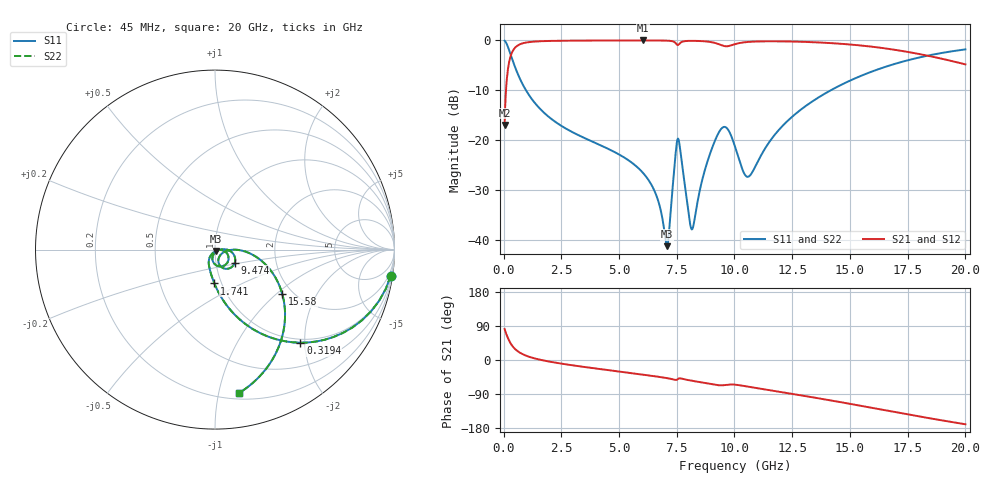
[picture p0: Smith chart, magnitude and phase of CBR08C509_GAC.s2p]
! S-parameter model data by Modelithics Inc.  support@modelithics.com 813-866-6335  Tampa FL USA
! S-Parameter data specifications:
! Substrate: 20-mil Rogers 4350B, substrate thickness, H=0.508mm, Dielectric constant, Er=3.75
! PCB Mounting Pad Footprint: Pad width, PadW=1.45mm , Pad length, PadL=1mm , Pad gap, PadG (edge-to-edge)=0.6mm , Reference planes=2.6mm apart
#  GHz  S  MA  R 50
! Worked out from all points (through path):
!   801 points, 45 MHz to 20 GHz, reference 50 ohm
!   highest |S21| = -0.04 dB at 6.032 GHz (marker M1); lowest = -17.0 dB at 45 MHz (marker M2)
!   group delay of S21, straight-line fit = 25.7 ps
!   lowest |S11| = -41.3 dB at 7.079 GHz (marker M3), VSWR 1.02, Z = 50.4 - j0.777 ohm
!   |S11| at or under -10 dB: 965.8 MHz to 14.18 GHz (13.22 GHz wide, 175 % of centre)
!   |S22| runs from -41.3 to -0.1 dB; largest |S21 - S12| = 0
!   S11 on the Smith chart (normalised r, x): 45 MHz: 1, -14; 319.4 MHz: 0.93, -1.91; 1.741 GHz: 0.93, -0.36; 9.474 GHz: 1.23, -0.19; 15.58 GHz: 1.76, -1.10; 20 GHz: 0.25, -1.15
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0.045  0.99 -8.4  0.1409 81.6  0.1409 81.6  0.99 -8.4
0.194662  0.8516 -33.0  0.5239 57.0  0.5239 57.0  0.8516 -33.0
0.319381  0.7041 -47.5  0.7097 42.5  0.7097 42.5  0.7041 -47.5
0.768369  0.3842 -72.7  0.9224 17.2  0.9224 17.2  0.3842 -72.7
1.741175  0.1885 -91.1  0.9808 -1.4  0.9808 -1.4  0.1885 -91.1
3.387462  0.1075 -106.7  0.9923 -17.5  0.9923 -17.5  0.1075 -106.7
6.0315  0.04686 -125.3  0.9955 -38.6  0.9955 -38.6  0.04686 -125.3
6.704981  0.02412 -123.9  0.9946 -44.3  0.9946 -44.3  0.02412 -123.9
7.079137  0.008583 -63.9  0.991 -47.9  0.991 -47.9  0.008583 -63.9
7.528125  0.1008 -46.9  0.8987 -51.3  0.8987 -51.3  0.1008 -46.9
7.6279  0.08705 -86.5  0.9292 -48.4  0.9292 -48.4  0.08705 -86.5
8.027  0.01727 -92.9  0.9858 -53.3  0.9858 -53.3  0.01727 -92.9
8.176663  0.01276 -47.5  0.9865 -54.9  0.9865 -54.9  0.01276 -47.5
8.800256  0.0578 1.7  0.9717 -61.6  0.9717 -61.6  0.0578 1.7
9.473738  0.1325 -34.0  0.885 -66.7  0.885 -66.7  0.1325 -34.0
10.0225  0.08566 -74.2  0.9143 -65.0  0.9143 -65.0  0.08566 -74.2
10.62115  0.04297 -35.8  0.9634 -70.7  0.9634 -70.7  0.04297 -35.8
11.84339  0.1201 -0.4  0.976 -82.9  0.976 -82.9  0.1201 -0.4
13.36496  0.2428 -11.0  0.9571 -98.2  0.9571 -98.2  0.2428 -11.0
15.58496  0.4498 -33.5  0.8805 -122.1  0.8805 -122.1  0.4498 -33.5
16.68248  0.5552 -45.5  0.8189 -134.3  0.8189 -134.3  0.5552 -45.5
20  0.8096 -80.4  0.5729 -169.6  0.5729 -169.6  0.8096 -80.4
